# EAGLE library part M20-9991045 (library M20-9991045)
M20: 10 Pos Plug SIL Straight 3mm THT Connector 6.1mm pin Gold Source: Datasheet
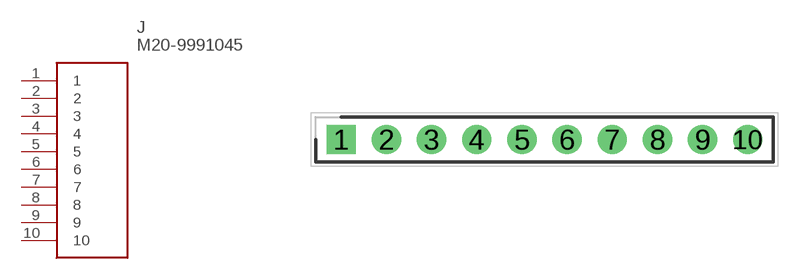
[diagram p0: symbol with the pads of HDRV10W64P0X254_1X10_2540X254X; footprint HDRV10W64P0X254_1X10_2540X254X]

Designator prefix J

## M20-9991045 (Description: M20: 10 Pos Plug SIL Straight 3mm THT Connector 6.1mm pin Gold; Height: 8.64mm; Manufacturer_Name: Harwin; Manufacturer_Part_Number: M20-9991045; Mouser_Part_Number: 855-M20-9991045; Mouser_Price-Stock: https://www.mouser.co.uk/ProductDetail/Harwin/M20-9991045?qs=%252Bk6%2F5FB6qrlmqe3AuAEP4g%3D%3D)  [HDRV10W64P0X254_1X10_2540X254X]
1  1
2  2
3  3
4  4
5  5
6  6
7  7
8  8
9  9
10  10

## Footprint HDRV10W64P0X254_1X10_2540X254X (pad centres in mm)
M20-9991045
drill 1.1 pad 1.65 square: 1 0,0
drill 1.1 pad 1.65: 2 2.54,0; 3 5.08,0; 4 7.62,0; 5 10.16,0; 6 12.7,0; 7 15.24,0; 8 17.78,0; 9 20.32,0; 10 22.86,0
